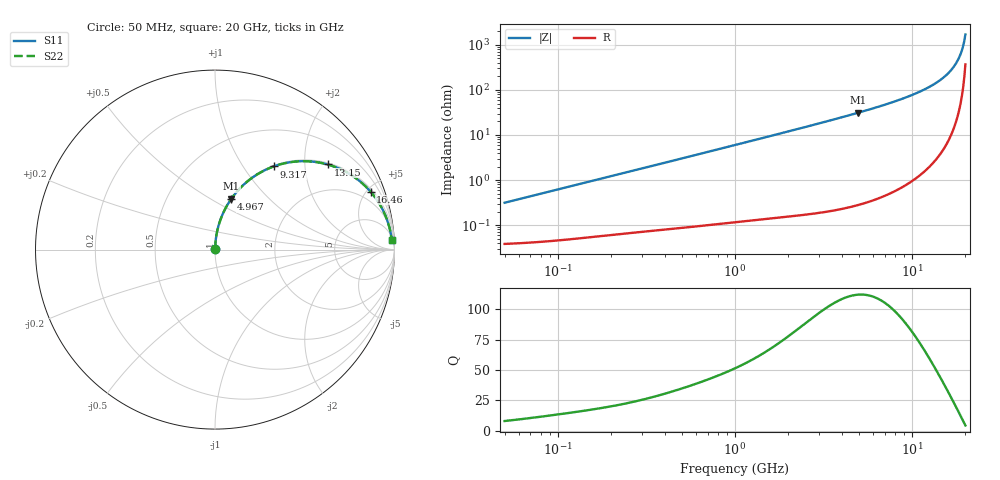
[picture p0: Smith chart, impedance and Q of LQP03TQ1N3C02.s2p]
!Murata Part Number: LQP03TQ1N3C02
!These Parameters are Measured in Series Mode Connection
!  o--[Z]--o
!Port1  Port2
!  o-------o
!Freq. Start=50[MHz] Stop=20[GHz], 401[Steps]
# Hz S RI R 50
!Freq.(Hz) S11(Real) S11(Imag) S21(Real) S21(Imag) S12(Real) S12(Imag) S22(Real) S22(Imag)
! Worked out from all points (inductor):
!   401 points, 50 MHz to 20 GHz, reference 50 ohm
!   read as one part in series: L = 989 pH near 51.52 MHz
!   highest Q = 112 at 4.967 GHz (marker M1), where L = 1 nH
!   S11 on the Smith chart (normalised r, x): 50 MHz: 1.00, +0.01; 4.967 GHz: 1.01, +0.63; 9.317 GHz: 1.02, +1.39; 13.15 GHz: 1.05, +2.61; 16.46 GHz: 1.19, +5.29; 20 GHz: 8, +33
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5e7  0.000392 0.00311  0.9996 -0.00311  0.9996 -0.00311  0.000392 0.00311
1.364002e8  0.000585 0.00838  0.9994 -0.00838  0.9994 -0.00838  0.000585 0.00838
3.721004e8  0.00127 0.0224  0.9987 -0.0224  0.9987 -0.0224  0.00127 0.0224
1e9  0.00473 0.0596  0.9953 -0.0596  0.9953 -0.0596  0.00473 0.0596
1.714689e9  0.0119 0.1014  0.9881 -0.1014  0.9881 -0.1014  0.0119 0.1014
2.728004e9  0.0281 0.1601  0.9719 -0.1601  0.9719 -0.1601  0.0281 0.1601
3.792786e9  0.0534 0.2201  0.9466 -0.2201  0.9466 -0.2201  0.0534 0.2201
4.966507e9  0.0912 0.2835  0.9088 -0.2835  0.9088 -0.2835  0.0912 0.2835
6.125241e9  0.1392 0.3417  0.8608 -0.3417  0.8608 -0.3417  0.1392 0.3417
7.442007e9  0.2069 0.4002  0.7931 -0.4002  0.7931 -0.4002  0.2069 0.4002
9.316812e9  0.3264 0.4632  0.6736 -0.4632  0.6736 -0.4632  0.3264 0.4632
1.131968e10  0.4787 0.4924  0.5213 -0.4924  0.5213 -0.4924  0.4787 0.4924
1.314879e10  0.6283 0.4741  0.3717 -0.4741  0.3717 -0.4741  0.6283 0.4741
1.482269e10  0.7591 0.4155  0.2409 -0.4155  0.2409 -0.4155  0.7591 0.4155
1.573793e10  0.8226 0.3675  0.1774 -0.3675  0.1774 -0.3675  0.8226 0.3675
1.646126e10  0.8668 0.3228  0.1332 -0.3228  0.1332 -0.3228  0.8668 0.3228
1.747767e10  0.9181 0.2518  0.0819 -0.2518  0.0819 -0.2518  0.9181 0.2518
1.828096e10  0.9488 0.191  0.0512 -0.191  0.0512 -0.191  0.9488 0.191
1.88369e10  0.9648 0.1476  0.0352 -0.1476  0.0352 -0.1476  0.9648 0.1476
1.912117e10  0.9712 0.1251  0.0288 -0.1251  0.0288 -0.1251  0.9712 0.1251
1.970266e10  0.9811 0.0791  0.0189 -0.0791  0.0189 -0.0791  0.9811 0.0791
2e10  0.9843 0.0556  0.0157 -0.0556  0.0157 -0.0556  0.9843 0.0556
